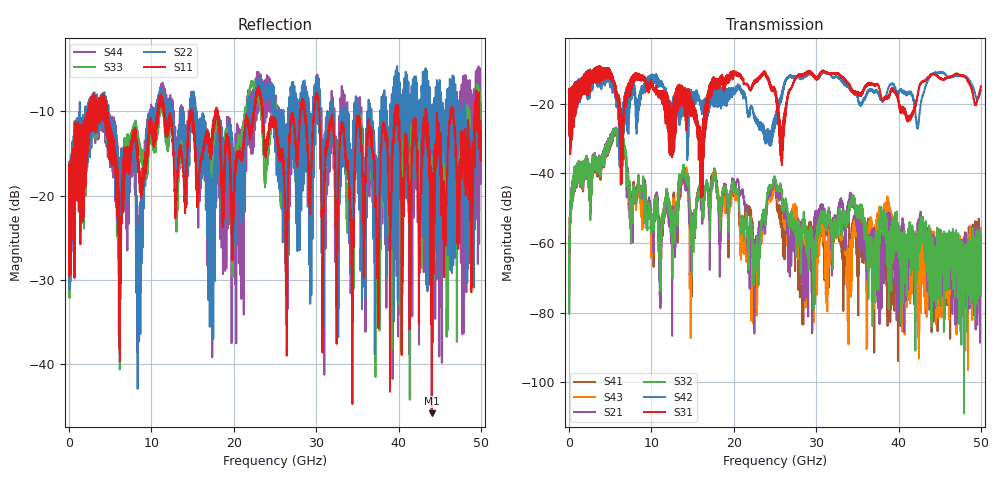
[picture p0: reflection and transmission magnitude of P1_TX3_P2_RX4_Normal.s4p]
!Keysight Technologies,N5225B,MY57041031,A.13.20.10
!Date: Friday, May 31, 2019 11:33:30
!Correction: S11(Full 4 Port(1,2,3,4))
!S12(Full 4 Port(1,2,3,4))
!S13(Full 4 Port(1,2,3,4))
!S14(Full 4 Port(1,2,3,4))
!S21(Full 4 Port(1,2,3,4))
!S22(Full 4 Port(1,2,3,4))
!S23(Full 4 Port(1,2,3,4))
!S24(Full 4 Port(1,2,3,4))
!S31(Full 4 Port(1,2,3,4))
!S32(Full 4 Port(1,2,3,4))
!S33(Full 4 Port(1,2,3,4))
!S34(Full 4 Port(1,2,3,4))
!S41(Full 4 Port(1,2,3,4))
!S42(Full 4 Port(1,2,3,4))
!S43(Full 4 Port(1,2,3,4))
!S44(Full 4 Port(1,2,3,4))
!S4P File: Measurements: <S11,S12,S13,S14>,
!<S21,S22,S23,S24>,
!<S31,S32,S33,S34>,
!<S41,S42,S43,S44>:
# Hz S  dB  R 50.0
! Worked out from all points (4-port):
!   5000 points, 10 MHz to 50 GHz, reference 50 ohm
!   strongest paths, dB at 10 MHz, 12.51 GHz, 25.01 GHz, 37.51 GHz, 50 GHz:
!     S31: -19.4, -27.2, -15.7, -14.5, -14.9
!     S42: -19.6, -27.2, -23.6, -16.9, -16.1
!     S32: -63.9, -56.5, -41.6, -67.0, -74.6
!     S21: -67.4, -66.9, -43.3, -63.1, -72.6
!     S43: -62.4, -52.6, -43.5, -51.6, -55.6
!     S41: -58.6, -54.2, -44.0, -59.5, -61.7
!   lowest |S11| = -45.9 dB at 44.03 GHz (marker M1), VSWR 1.01, Z = 49.9 + j0.505 ohm
!   |S11| at or under -10 dB: 4.66 GHz to 10.77 GHz (6.106 GHz wide, 79.2 % of centre); 23.49 GHz to 28.08 GHz (4.585 GHz wide, 17.8 % of centre); 30.37 GHz to 39.62 GHz (9.243 GHz wide, 26.4 % of centre)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
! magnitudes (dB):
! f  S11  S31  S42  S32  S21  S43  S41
! 10 MHz  -19.5  -19.4  -19.6  -63.9  -67.4  -62.4  -58.6
! 5.56 GHz  -16.0  -14.1  -14.6  -27.5  -27.5  -27.7  -28.2
! 11.12 GHz  -8.0  -17.3  -13.7  -72.4  -63.4  -63.2  -65.7
! 22.58 GHz  -8.9  -13.2  -24.2  -65.1  -62.9  -74.3  -60.9
! 24.95 GHz  -10.8  -15.8  -26.4  -41.3  -42.4  -42.8  -43.5
! 44.03 GHz  -45.9  -11.4  -11.6  -73.8  -64.1  -64.6  -70.0
! 50 GHz  -12.3  -14.9  -16.1  -74.6  -72.6  -55.6  -61.7
